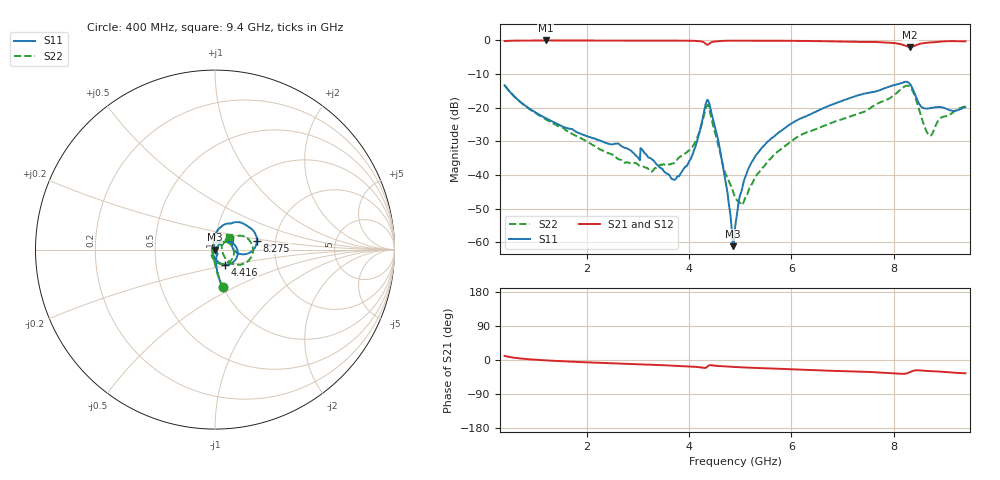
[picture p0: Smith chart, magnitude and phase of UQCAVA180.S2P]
!  Part Number  UQCAVA180 Mounting Orientation: Vertical
!  Description: RF capacitors
!  Application: Coupling, Bypass, Tuning, DC Block
!  Filters, Matching
# GHZ S DB R 50
! Freq  |S11|  S11 Ph  |S21|  S21 Ph  |S12|  S12 Ph  |S22|  S22 Ph
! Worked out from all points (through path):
!   801 points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, 400 MHz to 9.4 GHz, reference 50 ohm
!   highest |S21| = -0.06 dB at 1.199 GHz (marker M1); lowest = -2.0 dB at 8.32 GHz (marker M2)
!   group delay of S21, straight-line fit = 12.2 ps
!   lowest |S11| = -61.2 dB at 4.866 GHz (marker M3), VSWR 1.00, Z = 49.9 + j0.00562 ohm
!   |S11| at or under -10 dB: start of sweep to end of sweep
!   |S22| runs from -48.9 to -13.4 dB; largest |S21 - S12| = 0.0054
!   S11 on the Smith chart (normalised r, x): 400 MHz: 0.99, -0.44; 4.416 GHz: 1.10, -0.19; 8.275 GHz: 1.60, +0.17; 9.4 GHz: 1.18, +0.14
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0.4  -13.36 -78.8  -0.23 10.7  -0.21 10.7  -13.36 -78.7
1.199  -23.13 -85.1  -0.06 -1.0  -0.04 -1.0  -23.45 -92.7
1.908  -27.93 -77.3  -0.07 -5.6  -0.05 -5.7  -29.24 -109.3
2.999  -34.75 -57.3  -0.13 -11.2  -0.12 -11.2  -36.89 160.1
3.1  -32.77 -73.5  -0.12 -11.5  -0.11 -11.6  -37.52 -173.9
3.404  -37.31 -59.1  -0.09 -13.2  -0.07 -13.3  -37.49 -170.9
3.798  -40.38 3.8  -0.12 -15.4  -0.11 -15.5  -34.98 156.7
4.079  -33.58 45.5  -0.16 -17.5  -0.15 -17.6  -31.41 102.7
4.338  -18.40 5.7  -1.17 -19.9  -1.16 -20.1  -19.72 1.9
4.416  -19.97 -56.3  -0.80 -13.6  -0.79 -13.7  -21.65 -71.5
4.608  -32.58 -113.9  -0.25 -15.9  -0.24 -16.1  -33.27 -141.9
4.866  -61.16 176.3  -0.11 -18.2  -0.10 -18.4  -45.00 -169.5
4.9  -55.87 125.5  -0.11 -18.5  -0.10 -18.6  -46.66 -176.2
5.046  -43.61 114.7  -0.11 -19.4  -0.10 -19.6  -48.87 124.7
5.316  -34.00 106.9  -0.13 -21.0  -0.13 -21.1  -40.16 66.8
6.408  -21.73 88.8  -0.24 -26.6  -0.24 -26.8  -26.83 37.0
7.904  -13.81 48.3  -0.70 -34.3  -0.71 -34.5  -17.38 32.8
8.275  -12.43 12.1  -1.92 -34.5  -1.93 -34.7  -13.49 -3.4
8.32  -13.04 2.9  -2.04 -31.9  -2.05 -32.1  -13.88 -14.7
8.523  -19.44 -2.2  -1.02 -27.6  -1.04 -27.8  -21.89 -40.8
8.703  -20.21 16.6  -0.67 -29.3  -0.68 -29.5  -28.36 4.1
9.4  -19.84 34.2  -0.33 -35.0  -0.35 -35.2  -19.64 41.2
